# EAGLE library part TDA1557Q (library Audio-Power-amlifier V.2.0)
2 x 22 W BTL stereo car radio power amplifier with speaker protection
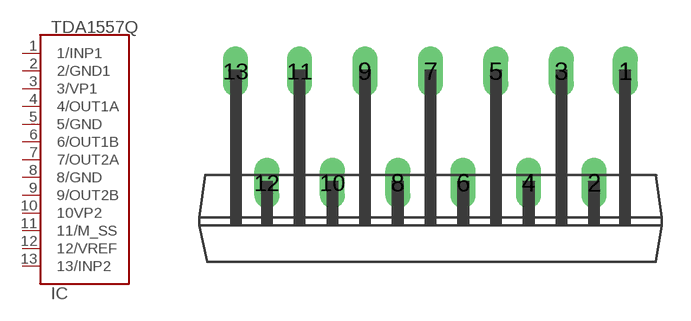
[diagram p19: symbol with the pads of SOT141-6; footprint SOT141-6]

Designator prefix IC

## TDA1557Q  [SOT141-6]
1  1/INP1  in
2  2/GND1  pwr
3  3/VP1  pwr
4  4/OUT1A  out
5  5/GND  pwr
6  6/OUT1B  out
7  7/OUT2A  out
8  8/GND  pwr
9  9/OUT2B  out
10  10VP2  pwr
11  11/M_SS  in
12  12/VREF  in
13  13/INP2  in

## Footprint SOT141-6 (pad centres in mm)
drill 0.8 long: 1 10.12,5.8; 2 8.5,0; 3 6.8,5.8; 4 5.1,0; 5 3.4,5.8; 6 1.7,0; 7 0,5.8; 8 -1.7,0; 9 -3.4,5.8; 10 -5.1,0; 11 -6.8,5.8; 12 -8.5,0; 13 -10.12,5.8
